FUNCTION_BLOCK FB_Mqtt
VAR CONSTANT
	cConnection : ST_ALYC_MqttConnectionSettings := (sHostName:='192.168.178.22', nHostPort:=1883, sClientId:='MyTestClient123', sUserID:='', sPassword:='');
	cConnection2 : ST_ALYC_MqttConnectionSettings := (sHostName:='192.168.178.89', nHostPort:=1883, sClientId:='MyTestClientNew', sUserID:='', sPassword:='');
//	cConnection:=(sHostName:='messagebroker.xyz.com', nHostPort:=8883,	bWithCertificate:=TRUE,
//	sCA:='C:\Users\xyz\Certs\CA_Cert.pem',
//	sCert:='C:\Users\xyz\Certs\ClientCert.pem',
//	sKey:= 'C:\Users\xyz\Certs\ClientKey.key'),

	cMqttTopic : STRING(255) :='Temp/TheNewTopic/PlcStreamX';
	cMqttTopic2 : STRING(255) :='Temp/TheNewTopic/PlcStreamX2';
	cMaxElements : UDINT := 40;
END_VAR
VAR
	// Stream
	fbMqttStream : FB_ALYC_MqttStream;	
	stMqttConfig: ST_ALYC_MqttStreamConfig := (
		bAutostartStream:=TRUE,
		nSamplingDivider:=2,
		nAdsBuffer:=40,
		stConnection:=cConnection,
		sMqttTopic:=cMqttTopic,
		stDeviceLocation:=(sAddress:= 'TheAddress', sLatitude:='TheLatitude', sLongitude:='TheLongitude'));

	stMqttConfig2: ST_ALYC_MqttStreamConfig := (
		bAutostartStream:=TRUE,
		nSamplingDivider:=1,
		nAdsBuffer:=10,
		stConnection:=cConnection2,
		sMqttTopic:=cMqttTopic,
		stDeviceLocation:=(sAddress:= 'TheNewAddress', sLatitude:='TheNewLatitude', sLongitude:='TheNewLongitude'));		
	
	bStart : BOOL := FALSE;
	bStop : BOOL := FALSE;
	bReconfigure : BOOL := FALSE;	
	bReconfigure2 : BOOL := FALSE;

	// StreamHelper
	fbMqttStreamHelper : FB_ALYC_MqttStreamHelper := (nObjectId := 16#01010010, nNumInputBuffer := cMaxElements);
	stMqttStreamHelperConfig: ST_ALYC_MqttStreamHelperConfig := (stConnection:=cConnection, sMqttTopic:=cMqttTopic);
	stMqttStreamHelperConfig2: ST_ALYC_MqttStreamHelperConfig := (stConnection:=cConnection2, sMqttTopic:=cMqttTopic);
		
	bReconfigureStreamHelper : BOOL := FALSE;	
	bReconfigureStreamHelper2 : BOOL := FALSE;	

	// Received 
	fbLrealSymbol : FB_ALYC_IotSymbol_LREAL := (stInitialConfig := (sSymbolName:='MAIN.fTest'));
	aLrealRcv : ARRAY[1..cMaxElements] OF LREAL;
	nElement : UDINT;
	nElementsReceived : ULINT;
END_VAR

// Stream
// Stream ist stopped by default and no topic is selected
// 1) Reconfigure stream
// 2) Start stream

// Stream
IF fbMqttStream.bInitialized THEN
	IF bStart THEN
		bStart := FALSE;
		fbMqttStream.Start();
	ELSIF bStop THEN
		bStop := FALSE;
		fbMqttStream.Stop();
	END_IF
	
	IF bReconfigure THEN	
		fbMqttStream.Reconfigure(stMqttConfig);
		IF fbMqttStream.eReconfigState = E_ALYC_ReconfigState.DONE THEN
			bReconfigure := FALSE;
		END_IF
	ELSIF bReconfigure2 THEN	
		fbMqttStream.Reconfigure(stMqttConfig2);
		IF fbMqttStream.eReconfigState = E_ALYC_ReconfigState.DONE THEN
			bReconfigure2 := FALSE;
		END_IF
	END_IF
END_IF

// StreamHelper
IF bReconfigureStreamHelper THEN
	fbMqttStreamHelper.Reconfigure(stMqttStreamHelperConfig);
	IF fbMqttStreamHelper.eReconfigState = E_ALYC_ReconfigState.DONE THEN
		bReconfigureStreamHelper := FALSE;
		fbMqttStreamHelper.AddIotSymbol(fbLrealSymbol);
	ELSE
		RETURN;
	END_IF
ELSIF bReconfigureStreamHelper2 THEN
	fbMqttStreamHelper.Reconfigure(stMqttStreamHelperConfig2);
	IF fbMqttStreamHelper.eReconfigState = E_ALYC_ReconfigState.DONE THEN
		bReconfigureStreamHelper2 := FALSE;
		fbMqttStreamHelper.AddIotSymbol(fbLrealSymbol);
	ELSE
		RETURN;
	END_IF
END_IF

IF NOT bReconfigureStreamHelper AND NOT bReconfigureStreamHelper2 THEN
	fbMqttStreamHelper.Call();
	FOR nElement := 1 TO fbMqttStreamHelper.nNumElements DO
		nElementsReceived := nElementsReceived + 1;
		aLrealRcv[nElement] := fbLrealSymbol.GetValue(nElement);
	END_FOR
END_IF

END_FUNCTION_BLOCK
